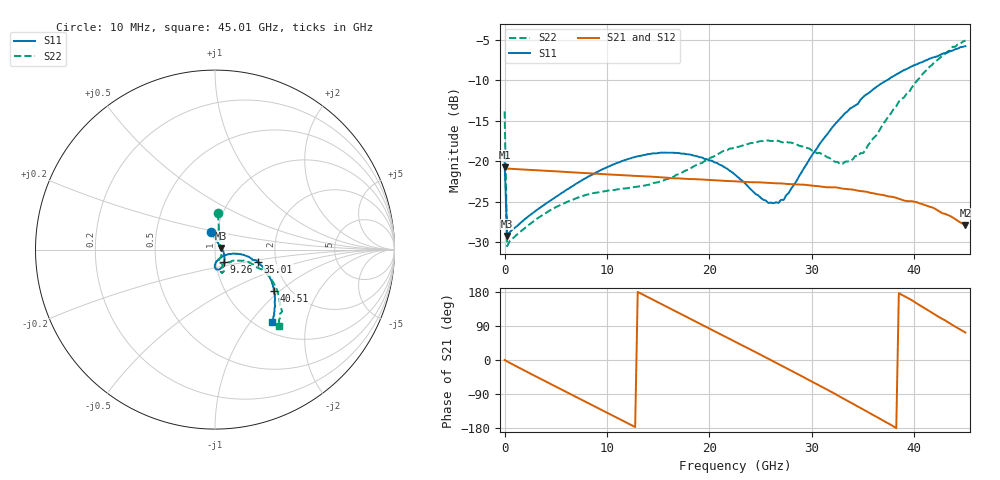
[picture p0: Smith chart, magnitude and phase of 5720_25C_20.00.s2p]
! Device:  ADRF5720
! Description: 0.5dB LSB GaAs MMIC 6-bit Digital Attenuator
! Frequency:  0.000009 -  40 GHz
! Ports:
!	RF1	= Port 1
!	RF2	= Port 2
! Vdd:  3.3 Volt
! Vss:  -3.3 Volt
! Control:  0/3.3 Volt
! State:  20.00 dB attenuation
! Data:  The device was measured using G-S-G Probes on a matrix board.
!  Data was collected using an calibrated 4 port network analyzer.
!  The reference plane for this measurement is at the launchers.
! Note:  Analog Devices supplies this data as a sample of measured data
!  for this product.  Your particular data for this product may vary.
!  Data was taken at 25 degrees C.
!  Analog Devices reserves the right to change this data at anytime.
# GHZ S DB R 45.0
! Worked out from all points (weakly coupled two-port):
!   181 points, 10 MHz to 45.01 GHz, reference 45 ohm
!   highest |S21| = -20.70 dB at 10 MHz (marker M1); lowest = -27.9 dB at 45.01 GHz (marker M2)
!   lowest |S11| = -29.2 dB at 260 MHz (marker M3), VSWR 1.07, Z = 48.1 + j0.867 ohm
!   |S11| at or under -10 dB: start of sweep to 37.33 GHz
!   |S22| runs from -30.5 to -5.1 dB; largest |S21 - S12| = 0.00021
!   S11 on the Smith chart (normalised r, x): 10 MHz: 0.94, +0.18; 9.26 GHz: 1.09, -0.16; 35.01 GHz: 1.61, -0.23; 40.51 GHz: 1.66, -0.92; 45.01 GHz: 1.17, -1.28
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0.01  -20.22 101.9  -20.70 -0.0  -20.70 -0.0  -13.84 85.3
0.26  -29.19 15.0  -20.89 -3.9  -20.90 -3.9  -30.46 15.1
0.51  -28.73 8.0  -20.91 -7.5  -20.92 -7.5  -29.82 5.7
3.26  -25.90 -17.7  -21.11 -46.0  -21.11 -46.0  -26.99 -35.0
7.76  -22.18 -47.2  -21.43 -108.1  -21.43 -108.1  -24.22 -68.3
9.26  -21.18 -54.6  -21.55 -128.7  -21.55 -128.7  -23.81 -73.1
12.51  -19.54 -68.5  -21.78 -173.5  -21.78 -173.4  -23.20 -75.2
15.26  -18.93 -78.3  -21.95 148.4  -21.95 148.4  -22.45 -70.1
19.26  -19.51 -88.6  -22.24 93.2  -22.24 93.2  -20.22 -63.5
21.26  -20.53 -90.4  -22.38 65.6  -22.39 65.6  -18.79 -64.1
22.76  -21.92 -89.4  -22.48 44.9  -22.48 45.0  -18.24 -65.8
25.26  -24.73 -70.4  -22.61 10.3  -22.61 10.3  -17.50 -70.6
26.76  -25.13 -46.2  -22.71 -10.6  -22.71 -10.6  -17.48 -72.4
27.76  -23.89 -29.2  -22.80 -24.7  -22.80 -24.6  -17.68 -74.2
30.26  -18.82 -11.3  -23.02 -60.4  -23.02 -60.4  -18.75 -73.5
32.76  -14.78 -11.7  -23.30 -96.8  -23.30 -96.8  -20.33 -59.7
35.01  -12.09 -16.0  -23.70 -130.0  -23.71 -130.0  -18.99 -34.5
37.76  -9.64 -25.4  -24.36 -171.6  -24.36 -171.6  -14.06 -20.4
40.51  -7.88 -35.2  -25.17 145.2  -25.17 145.2  -9.75 -25.9
42.26  -7.05 -41.5  -26.01 116.0  -26.01 115.9  -7.52 -33.9
43.76  -6.34 -46.9  -26.91 92.1  -26.91 92.2  -5.87 -42.7
45.01  -5.79 -52.0  -27.91 72.5  -27.91 72.5  -5.09 -50.1
